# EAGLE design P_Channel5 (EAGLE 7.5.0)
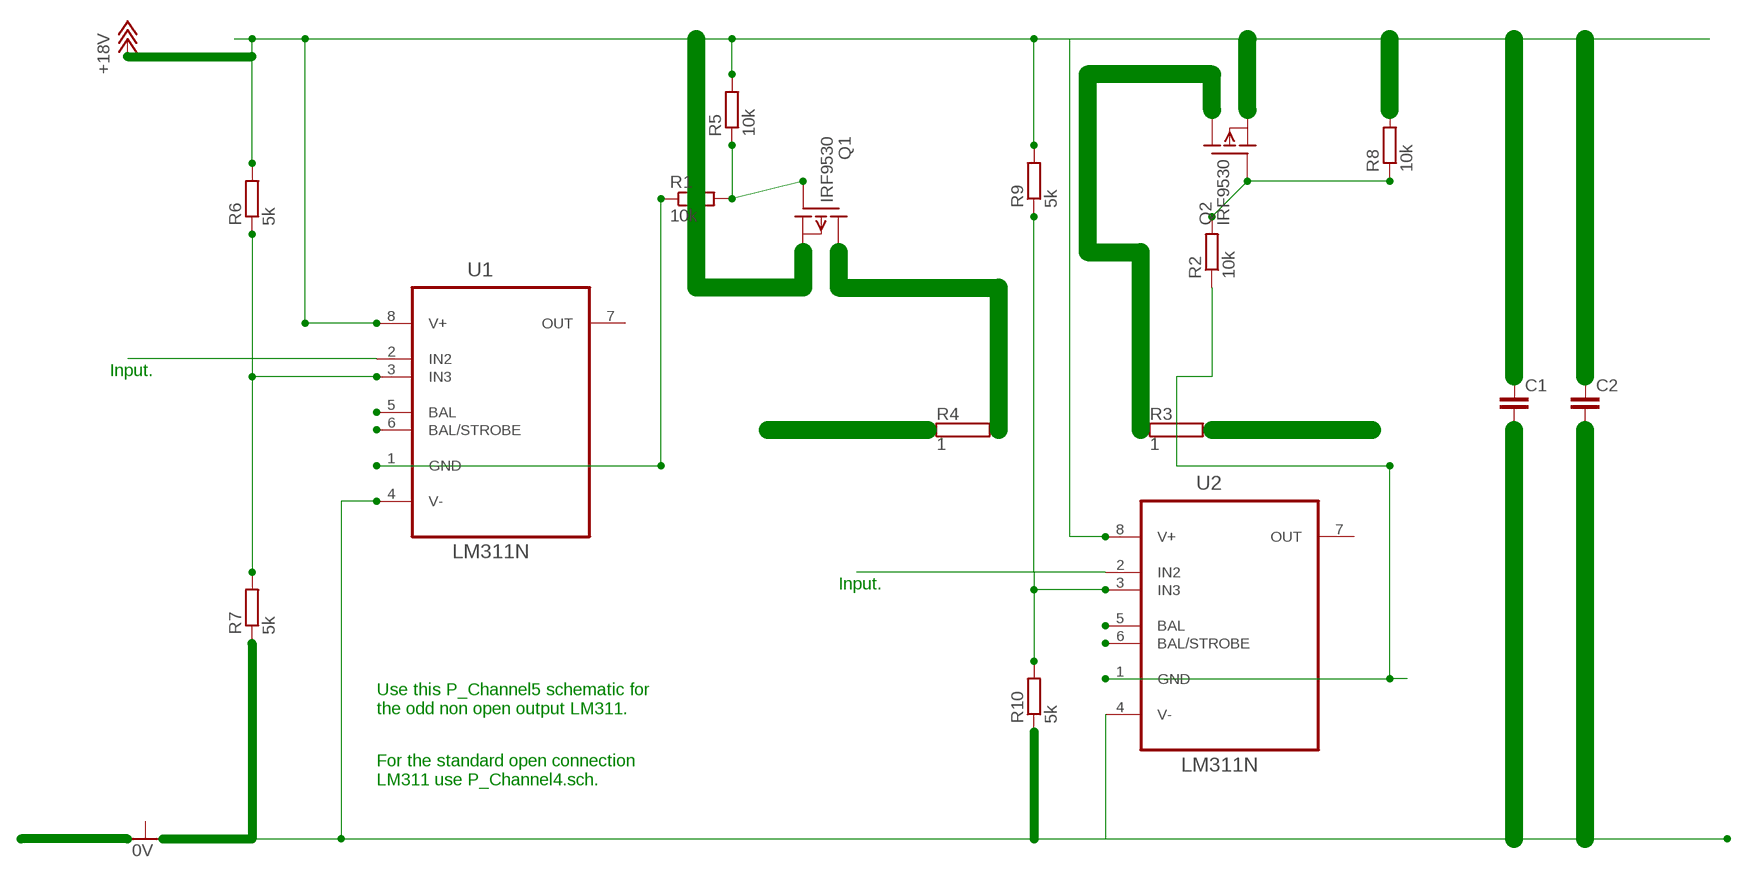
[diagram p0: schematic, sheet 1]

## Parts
C1  C7.5/3  [C7.5B3]
C2  C7.5/3  [C7.5B3]
Q1  IRF9530  [TO220]
Q2  IRF9530  [TO220]
R1  10k  R-EU_0207/10  [0207/10]
R2  10k  R-EU_0207/10  [0207/10]
R3  1  RMG100-H  [TO-247-2H]
R4  1  RMG100-H  [TO-247-2H]
R5  10k  R-EU_0207/10  [0207/10]
R6  5k  R-EU_0207/10  [0207/10]
R7  5k  R-EU_0207/10  [0207/10]
R8  10k  R-EU_0207/10  [0207/10]
R9  5k  R-EU_0207/10  [0207/10]
R10  5k  R-EU_0207/10  [0207/10]
U1  LM311N  [DIP254P762X508-8]
U2  LM311N  [DIP254P762X508-8]

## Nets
+18V: C1.1 C1.2 C2.1 C2.2 Q1.3(S) Q2.3(S) R5.2 R6.2 R7.1 R9.2 R10.1 U1.4(V-) U1.8(V+) U2.4(V-) U2.8(V+)
N$1: Q1.1(G) R1.2 R5.1
N$2: Q2.1(G) R2.2 R8.1
N$4: Q2.2(D) R3.1
N$5: U1.5(BAL)
N$6: R1.1 U1.1(GND)
N$7: Q1.2(D) R2.1 R3.2 R4.1 R4.2 U2.1(GND)
N$8: R6.1 R7.2 R9.1 R10.2 U1.3(IN3) U2.3(IN3)
N$9: U1.2(IN2)
N$10: U2.2(IN2)
N$11: U1.6(BAL/STROBE)
N$12: U2.5(BAL)
N$13: U2.6(BAL/STROBE)
Unconnected: R8.2 U1.7(OUT) U2.7(OUT)

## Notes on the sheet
- Input.
- Input.
- Use this P_Channel5 schematic for 
  the odd non open output LM311.
- For the standard open connection
  LM311 use P_Channel4.sch.

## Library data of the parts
C1 C2 = capacitor-wima:C: CAPACITOR
Q1 Q2 = transistor-fet:IRF9530: P-Channel Enhancement MOSFET (HEXFET); -100V; -12A; 0,3Ohm
R1 R2 R5-R10 = rcl:R-EU_: RESISTOR, European symbol
R3 R4 = resistor-power:RMG100: TO-247 Power Resistor - RMG 100 Series; OC_FARNELL: unknown; OC_NEWARK: unknown
U1 U2 = NSC_By_element14_Batch_1.1:LM311N: Voltage Comparator; MPN: LM311N; OC_FARNELL: 9487220; OC_NEWARK: 07B6414; PACKAGE: DIP-8; SUPPLIER: NationalSemiconductor

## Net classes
0 default: clearance 0.205 mm

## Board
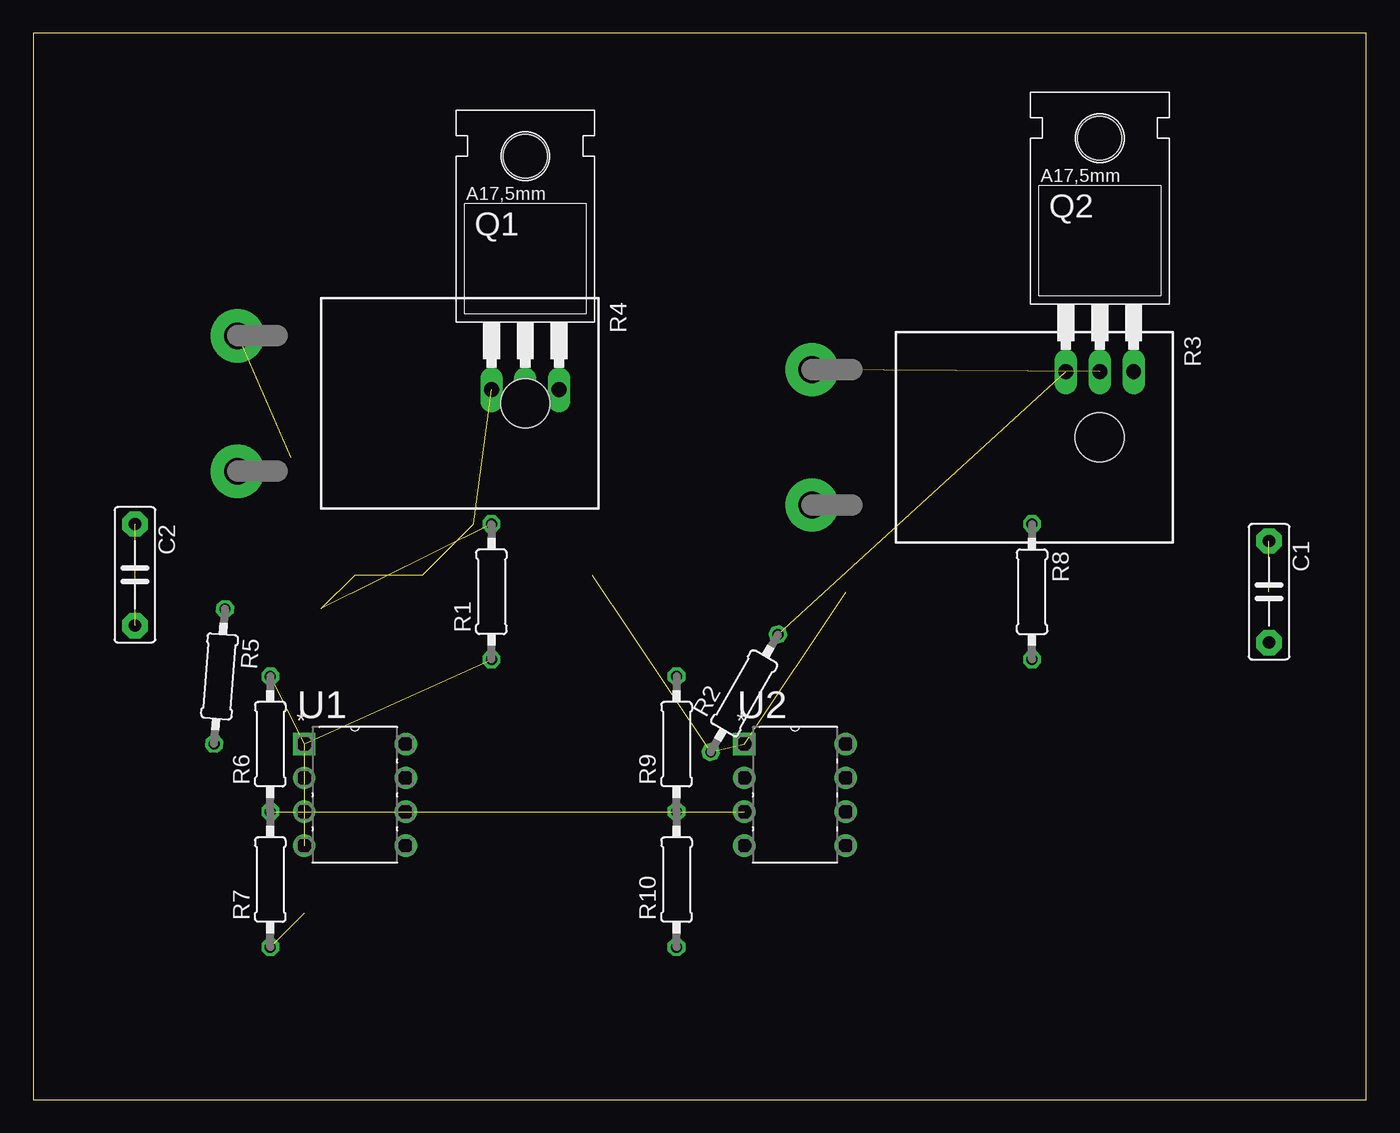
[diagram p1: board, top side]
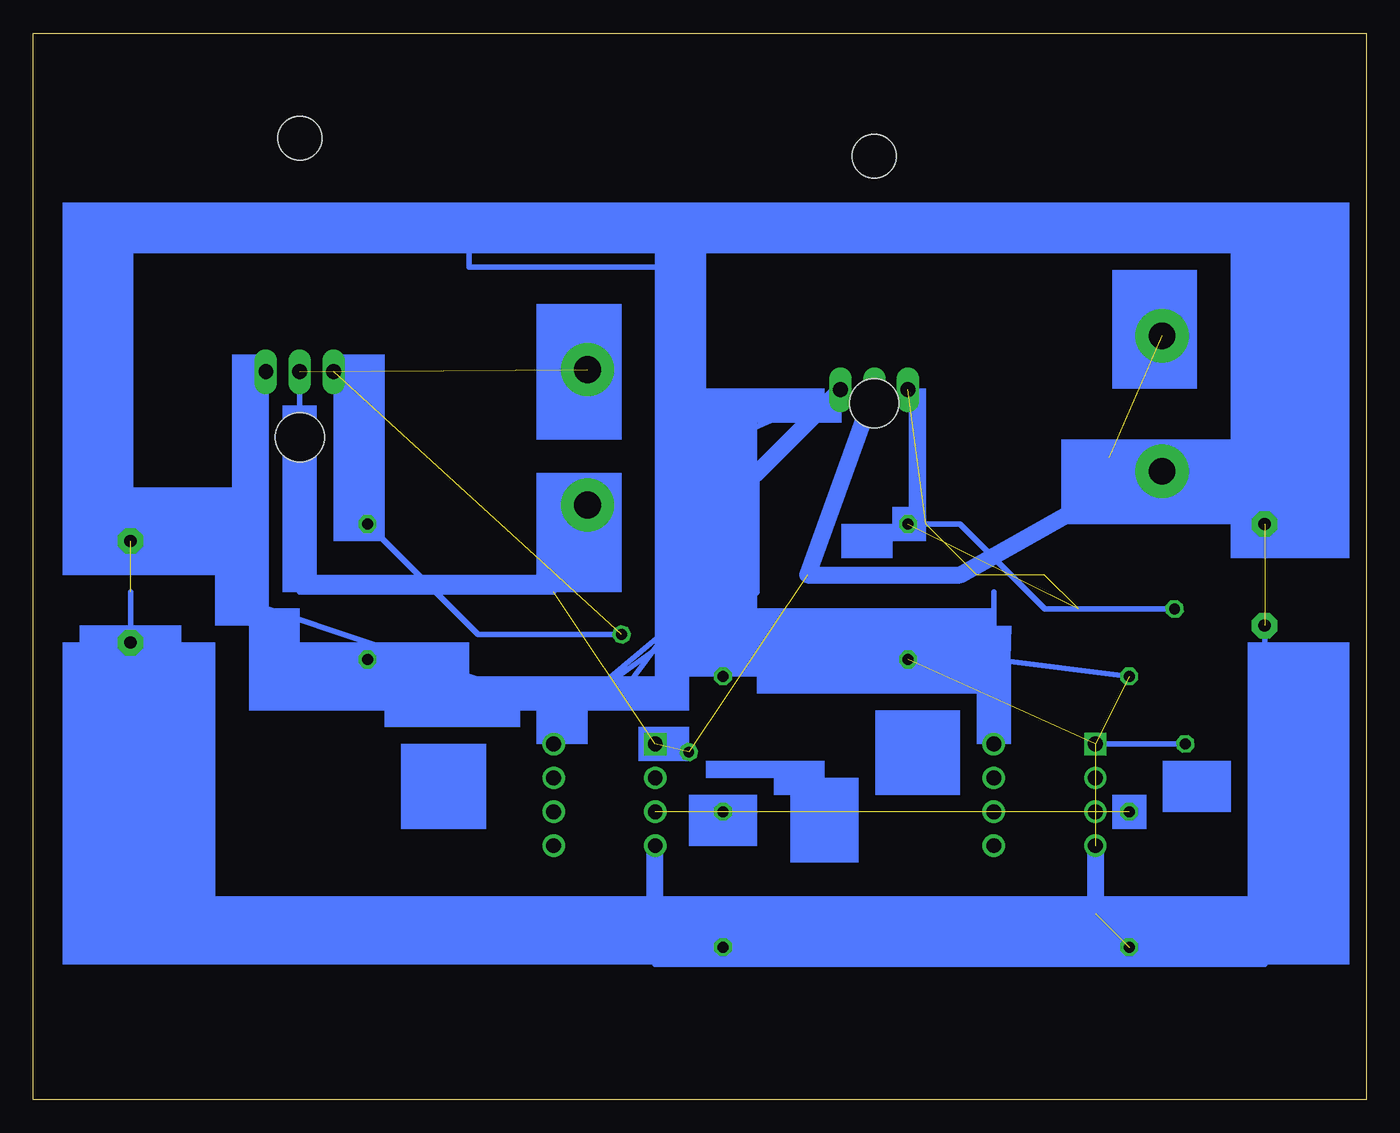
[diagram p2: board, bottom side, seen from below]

Size 100 x 80 mm. Coordinates in mm from the lower left corner, seen from the top.
Outline: 0,0 100,0 100,80 0,80 0,0
Copper layers (1*16): Top 0.035mm / dielectric 1.5mm / Bottom 0.035mm
Design rules "default": minimum track width 10mil, minimum drill 24mil, track to track 8mil, track to pad 8mil, pad to pad 8mil, via to via 8mil, smd to smd 8mil, copper to edge 40mil, drill to drill 8mil, minimum pad ring 10mil, minimum via ring 8mil, stop-mask expansion 4mil, vias tented up to drill 0mil, thermal gap 10mil

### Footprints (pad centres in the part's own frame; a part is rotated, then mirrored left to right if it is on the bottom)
C7.5B3 = drill 0.914 pad 1.905 octagon: 1 -3.81,0; 2 3.81,0
TO220 = drill 1.118 long: 1 -2.54,-6.35; 2 0,-6.35; 3 2.54,-6.35 | hole 3.302: 0,11.176
0207/10 = drill 0.813 octagon: 1 -5.08,0; 2 5.08,0
TO-247-2H = drill 2 pad 4: 1 -5.08,-21.59; 2 5.08,-21.59 | hole 3.7: 0,0
DIP254P762X508-8 = drill 1.118 square: 1 -7.62,7.62 | drill 1.118: 2 -7.62,5.08; 3 -7.62,2.54; 4 -7.62,0; 5 0,0; 6 0,2.54; 7 0,5.08; 8 0,7.62

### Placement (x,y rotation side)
C1  92.71,38.1 270 top
C2  7.62,39.37 270 top
Q1  36.91,59.61 0 top
Q2  80.01,60.96 0 top
R1  34.37,38.1 90 top
R2  53.34,30.48 60.3 top
R3  80.01,49.69 270 top
R4  36.91,52.23 270 top
R5  13.97,31.75 265.4 top
R6  17.78,26.67 90 top
R7  17.78,16.51 90 top
R8  74.93,38.1 270 top
R9  48.26,26.67 90 top
R10  48.26,16.51 90 top
U1  27.94,19.05 0 top
U2  60.96,19.05 0 top

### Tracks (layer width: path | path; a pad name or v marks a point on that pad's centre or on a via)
+18V  (5 unrouted)
  Bottom 0.406: 92.71,38.1 C1.2 92.71,12.7 53.34,12.7 | C1.1 92.71,45.72 | 92.71,45.72 92.71,63.74 67.31,63.74 67.31,62.47 50.8,62.47 50.8,48.26 | C2.2 7.62,10.16 13.97,10.16 | 13.97,10.16 53.34,10.16 53.34,12.7 | R7.1 13.97,10.16 | 27.94,33.02 U1.8 | R6.2 27.94,33.02 | 27.94,33.02 27.94,38.1 | 45.72,46.99 45.72,38.1 48.26,35.56 R9.2 50.8,35.56 | U2.8 60.96,27.94 59.69,29.21 | 59.69,29.21 55.88,30.48 52.07,35.56 59.69,29.21 | 59.69,29.21 82.55,36.83 82.55,45.72 | 82.55,45.72 Q2.3 | 59.69,29.21 50.8,35.56 | 53.34,12.7 R10.1 | 82.55,45.72 92.71,45.72 | Q1.3 50.8,48.26 | 50.8,48.26 50.8,35.56 | R5.2 20.3,26.69 | 20.32,13.97 21.59,12.7
  Bottom 1.27: 53.34,12.7 U2.4 | 45.72,46.99 Q1.3 | U1.4 20.32,13.97
N$1  (5 unrouted)
  Bottom 0.406: R5.1 24.11,36.81 30.48,43.18 R1.2
N$2  (1 unrouted)
  Bottom 0.406: R2.2 66.64,34.89 R8.1
N$4  (1 unrouted)
N$6  (1 unrouted)
N$7  (4 unrouted)
  Bottom 0.406: 19.29,45.64 19.29,48.18 R4.2 | R3.2 60.96,38.1 80.01,38.1 80.01,54.61
  Bottom 1.27: Q1.2 41.91,39.37 30.48,39.37 19.29,45.64
N$8  (3 unrouted)
(copper drawn outside any net)
  shapes: Bottom area x74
